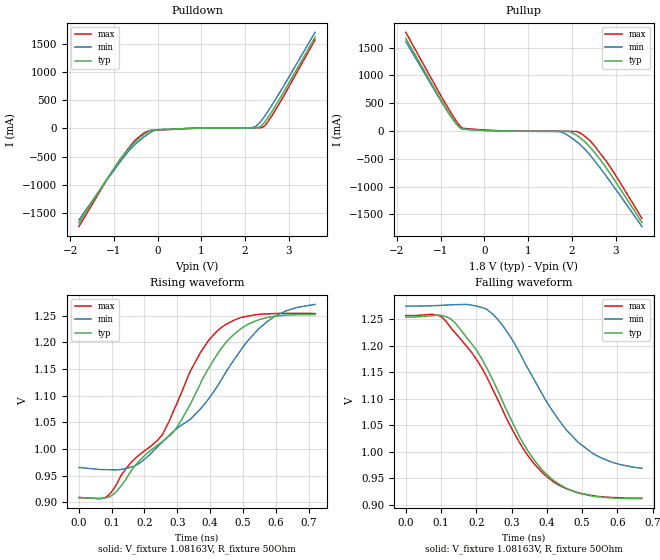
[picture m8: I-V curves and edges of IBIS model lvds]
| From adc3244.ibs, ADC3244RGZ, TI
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|   lvds Model
[Model]   lvds
Model_type   Output
Polarity   Non-Inverting
Vmeas = 1.08163
Vref = 1.08163
Cref = 5pF
Rref = 50
|   typ   min   max
|   (nom PVT)   (fast PVT)   (slow PVT)
C_comp   2.093e-12   2.051e-12   2.106e-12
| Where nom  PVT is Nominal Process, 1.8V, 27C
|   Fast PVT is Strong Process,  1.9V, -40C
|   Slow PVT is Weak Process,   1.7V, 125C
[Voltage Range]   1.8   1.7   1.9
|Junction Temperature
[Temperature Range]   27   125   -40
[Pullup Reference]   1.8   1.7   1.9
[Pulldown Reference]   0   0   0
[Power Clamp Reference]   1.8   1.7   1.9
[GND Clamp Reference]   0   0   0
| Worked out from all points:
|   slope of the pulldown table from 0 to 0.27 V, typ, clamps not added: 31.2 ohm
|   slope of the pullup table from 0 to 0.27 V, typ, clamps not added: 30.3 ohm
|   falling waveform, V_fixture 1.08163V, R_fixture 50Ohm: 20-80 % time 163ps typ, 171ps min, 173ps max; typ from 1.25 V to 0.911 V
|   rising waveform, V_fixture 1.08163V, R_fixture 50Ohm: 20-80 % time 244ps typ, 248ps min, 211ps max; typ from 0.909 V to 1.25 V
[Pulldown]
|   Voltage   I(typ)   I(min)   I(max)
-1.8V     -1.68A     -1.629A    -1.746A
-874.7mV  -574.7mA   -613.1mA   -570.8mA
-511.2mV  -235mA     -280.3mA   -209.8mA
-300.9mV  -100.6mA   -145.9mA   -74.97mA
-162mV    -38.5mA    -71.3mA    -35.7mA
24.1mV    -25.19mA   -20.26mA   -30.06mA
1.982V    6.103mA    5.447mA    5.623mA
2.236V    10.43mA    32.17mA    7.801mA
2.322V    21.08mA    91.3mA     10.4mA
2.429V    91.8mA     197.7mA    33.86mA
2.61V     294.9mA    409.2mA    220.6mA
3.6V      1.622A     1.709A     1.575A
[Pullup]
|   Voltage   I(typ)   I(min)   I(max)
-1.8V     1.666A     1.61A      1.773A
-819.1mV  332.1mA    319.2mA    395.8mA
-644.4mV  129.1mA    127.9mA    176.4mA
-540.3mV  48.29mA    49.99mA    72.14mA
-487.1mV  34.08mA    31.12mA    46.59mA
250.2mV   2.569mA    -4.165uA   6.609mA
1.716V    -7.035mA   -13.25mA   -6.789mA
1.976V    -20.79mA   -117.1mA   -7.257mA
2.194V    -129.8mA   -250.6mA   -40.14mA
2.426V    -303mA     -444.9mA   -187.1mA
2.781V    -661.5mA   -810.9mA   -541mA
3.6V      -1.646A    -1.72A     -1.575A
[Ramp]
R_load = 50
|   typ   min   max
dV/dt_r   0.0858516/4.21677e-11   0.0237527/3.76052e-11 0.107974/3.52289e-11
dV/dt_f   0.206308/1.32611e-10   0.18671/1.50587e-10   0.208145/1.33412e-10
[Falling Waveform]
V_fixture = 1.08163V
V_fixture_min = 1.11877V
V_fixture_max = 1.08292V
R_fixture = 50Ohm
|   Time   V(typ)   V(min)   V(max)
0s        1.254V     1.274V     1.257V
92ps      1.258V     1.276V     1.257V
126ps     1.251V     1.277V     1.235V
230ps     1.158V     1.268V     1.141V
276ps     1.093V     1.237V     1.077V
334ps     1.015V     1.173V     1.005V
418ps     946.2mV    1.075V     943.5mV
460ps     929.3mV    1.038V     928.9mV
528ps     916.2mV    997.9mV    917mV
670ps     911.1mV    968.6mV    911.9mV
[Rising Waveform]
V_fixture = 1.08163V
V_fixture_min = 1.11877V
V_fixture_max = 1.08292V
R_fixture = 50Ohm
|   Time   V(typ)   V(min)   V(max)
0s        909.2mV    965.6mV    909mV
98ps      912.2mV    961.1mV    918.5mV
174ps     970.7mV    969.5mV    983.7mV
252ps     1.013V     1.011V     1.025V
298ps     1.04V      1.038V     1.085V
368ps     1.119V     1.074V     1.178V
436ps     1.19V      1.132V     1.229V
506ps     1.231V     1.196V     1.248V
574ps     1.247V     1.239V     1.253V
720ps     1.252V     1.271V     1.254V
